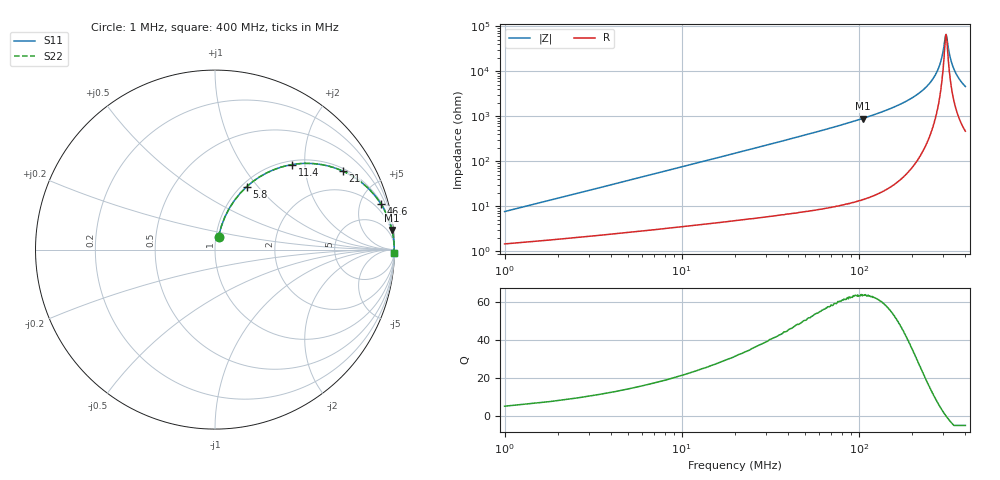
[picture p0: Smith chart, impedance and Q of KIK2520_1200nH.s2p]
!version-2
!date-01.2022
!Series
# MHz S RI R 50
!Freq ReS11 ImS11 ReS21 ImS21 ReS12 ImS12 ReS22 ImS22
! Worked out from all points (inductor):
!   500 points, 1 MHz to 400 MHz, reference 50 ohm
!   read as one part in series: L = 1.2 uH near 2.6 MHz
!   highest Q = 63.6 at 105 MHz (marker M1), where L = 1.35 uH
!   self-resonance near 311 MHz
!   S11 on the Smith chart (normalised r, x): 1 MHz: 1.03, +0.15; 5.8 MHz: 1.06, +0.87; 11.4 MHz: 1.07, +1.72; 21 MHz: 1.10, +3.18; 46.6 MHz: 1.15, +7.19; 400 MHz: 10, -91
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1  0.0199 0.0728  0.9801 -0.0728  0.9801 -0.0728  0.0199 0.0728
3.4  0.08 0.2306  0.92 -0.2306  0.92 -0.2306  0.08 0.2306
5.8  0.1764 0.3504  0.8236 -0.3504  0.8236 -0.3504  0.1764 0.3504
11.4  0.4291 0.4737  0.5709 -0.4737  0.5709 -0.4737  0.4291 0.4737
21  0.711 0.4381  0.289 -0.4381  0.289 -0.4381  0.711 0.4381
31.4  0.8452 0.3495  0.1548 -0.3495  0.1548 -0.3495  0.8452 0.3495
46.6  0.9237 0.2554  0.0763 -0.2554  0.0763 -0.2554  0.9237 0.2554
68.2  0.964 0.1778  0.036 -0.1778  0.036 -0.1778  0.964 0.1778
105  0.9859 0.1101  0.0141 -0.1101  0.0141 -0.1101  0.9859 0.1101
134  0.9922 0.08  0.00779 -0.08  0.00779 -0.08  0.9922 0.08
201  0.9974 0.0383  0.00257 -0.0383  0.00257 -0.0383  0.9974 0.0383
239  0.9983 0.0228  0.00169 -0.0228  0.00169 -0.0228  0.9983 0.0228
267  0.9986 0.0132  0.00145 -0.0132  0.00145 -0.0132  0.9986 0.0132
291  0.9986 0.00577  0.00143 -0.00577  0.00143 -0.00577  0.9986 0.00577
299  0.9985 0.00346  0.00145 -0.00346  0.00145 -0.00346  0.9985 0.00346
308  0.9985 0.00077  0.0015 -0.00077  0.0015 -0.00077  0.9985 0.00077
311  0.9985 0.000111  0.00152 -0.000111  0.00152 -0.000111  0.9985 0.000111
315  0.9985 -0.000976  0.00154 0.000976  0.00154 0.000976  0.9985 -0.000976
324  0.9984 -0.00353  0.00162 0.00353  0.00162 0.00353  0.9984 -0.00353
334  0.9983 -0.00601  0.00171 0.00601  0.00171 0.00601  0.9983 -0.00601
360  0.998 -0.0125  0.00203 0.0125  0.00203 0.0125  0.998 -0.0125
400  0.9973 -0.0215  0.00268 0.0215  0.00268 0.0215  0.9973 -0.0215
